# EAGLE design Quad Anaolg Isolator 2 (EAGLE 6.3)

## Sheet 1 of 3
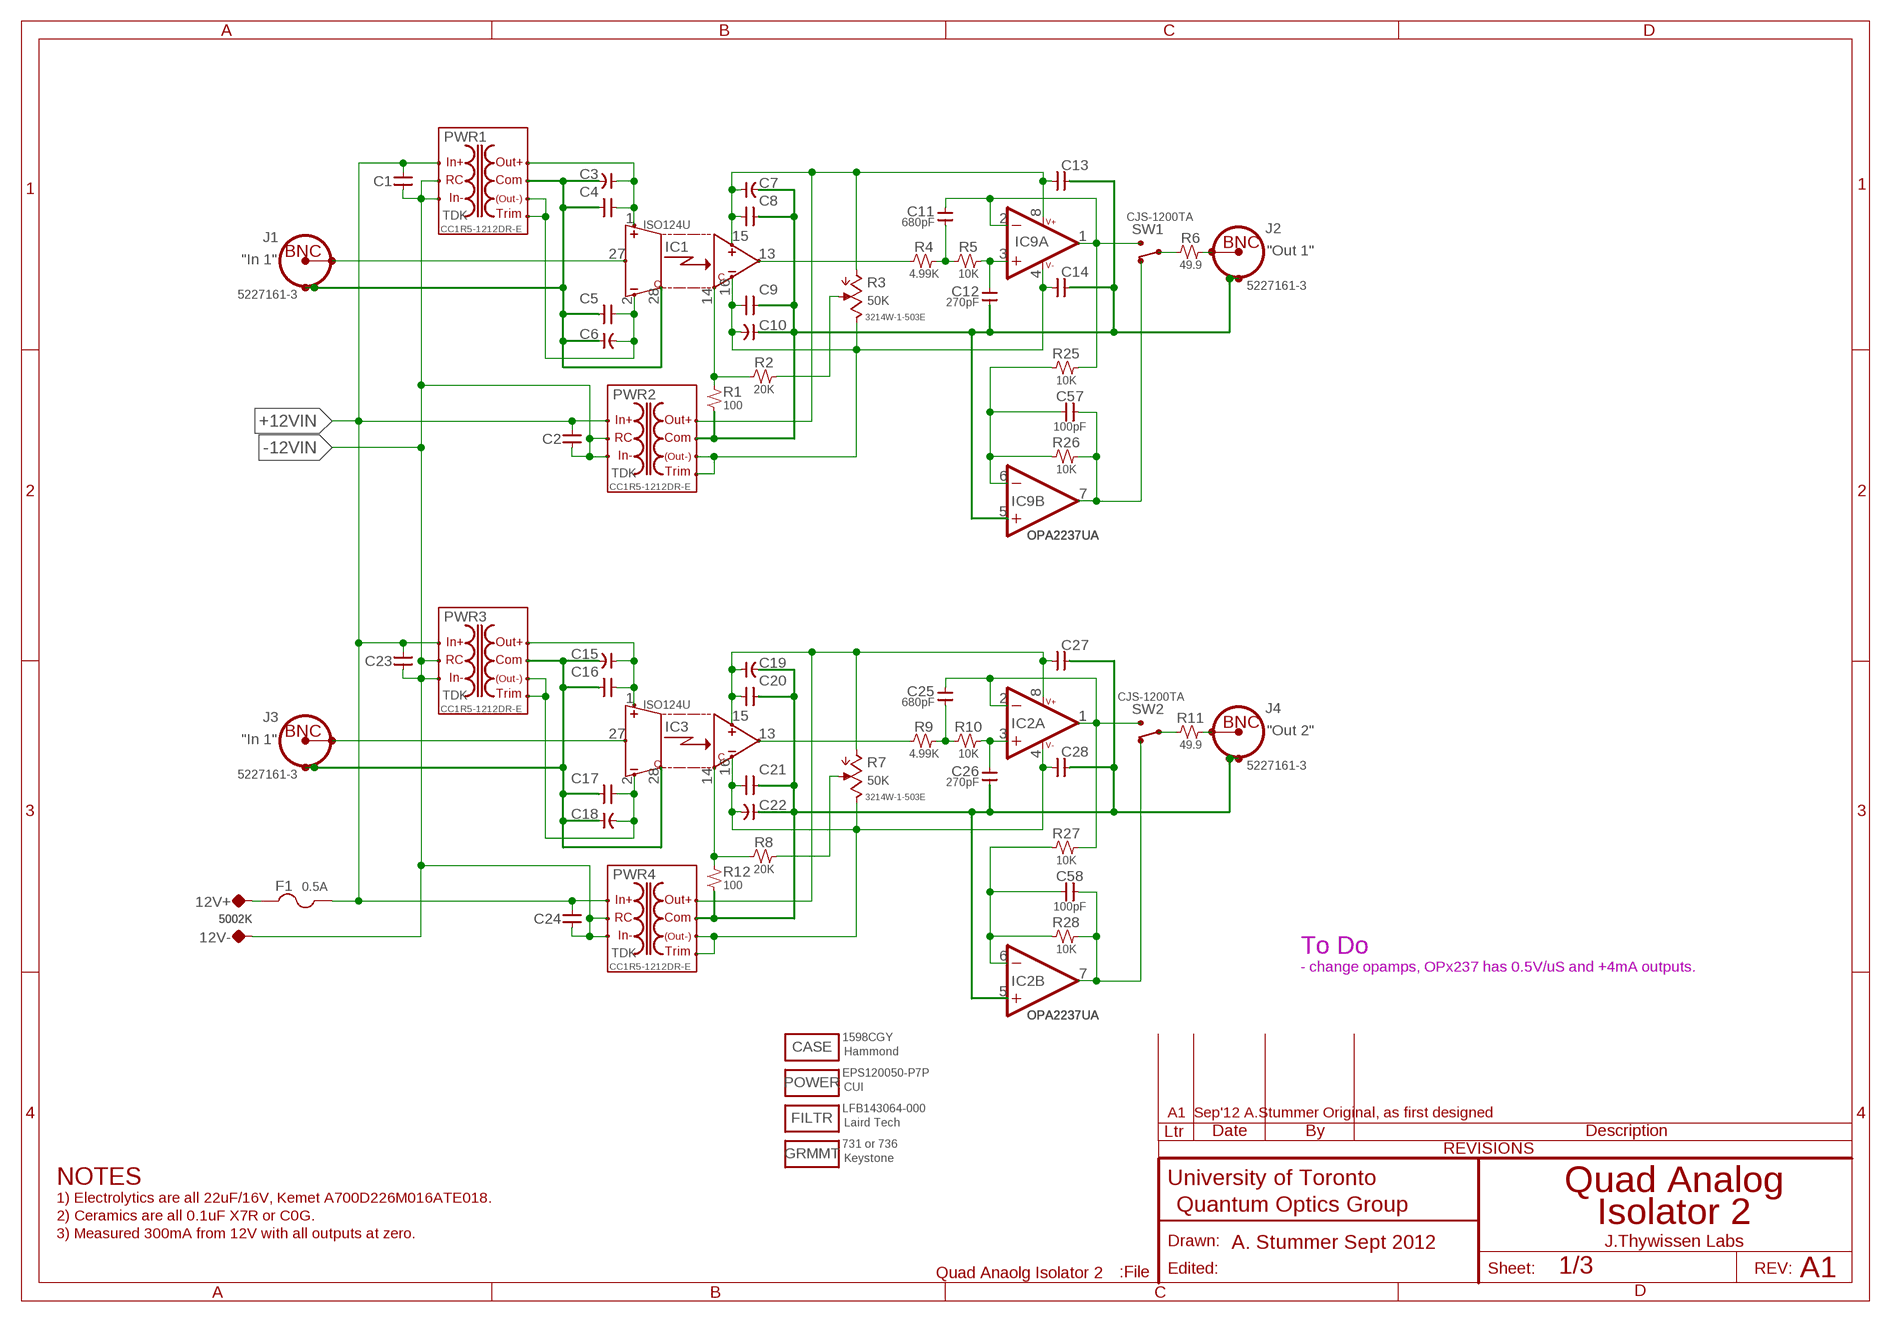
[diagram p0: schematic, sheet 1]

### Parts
12V+  5002K  TP-0.042B  [TP-0.042B]
12V-  5002K  TP-0.042B  [TP-0.042B]
C1  0.1uF  CAP-H-0805  [2012(0805)]
C2  0.1uF  CAP-H-0805  [2012(0805)]
C3  22uF  CAP-POL-2917(7343)  [2917(7343)]
C4  0.1uF  CAP-H-0805  [2012(0805)]
C5  0.1uF  CAP-H-0805  [2012(0805)]
C6  22uF  CAP-POL-2917(7343)  [2917(7343)]
C7  22uF  CAP-POL-2917(7343)  [2917(7343)]
C8  0.1uF  CAP-H-0805  [2012(0805)]
C9  0.1uF  CAP-H-0805  [2012(0805)]
C10  22uF  CAP-POL-2917(7343)  [2917(7343)]
C11  680pF  CAP-V-0805  [2012(0805)]
C12  270pF  CAP-V-0805  [2012(0805)]
C13  0.1uF  CAP-H-0805  [2012(0805)]
C14  0.1uF  CAP-H-0805  [2012(0805)]
C15  22uF  CAP-POL-SMT,8MM,PLASTIC_BASE  [CAP,POL,8MM,PLASTIC_BASE]
C16  0.1uF  CAP-H-0805  [2012(0805)]
C17  0.1uF  CAP-H-0805  [2012(0805)]
C18  22uF  CAP-POL-SMT,8MM,PLASTIC_BASE  [CAP,POL,8MM,PLASTIC_BASE]
C19  22uF  CAP-POL-SMT,8MM,PLASTIC_BASE  [CAP,POL,8MM,PLASTIC_BASE]
C20  0.1uF  CAP-H-0805  [2012(0805)]
C21  0.1uF  CAP-H-0805  [2012(0805)]
C22  22uF  CAP-POL-SMT,8MM,PLASTIC_BASE  [CAP,POL,8MM,PLASTIC_BASE]
C23  0.1uF  CAP-H-0805  [2012(0805)]
C24  0.1uF  CAP-H-0805  [2012(0805)]
C25  680pF  CAP-V-0805  [2012(0805)]
C26  270pF  CAP-V-0805  [2012(0805)]
C27  0.1uF  CAP-H-0805  [2012(0805)]
C28  0.1uF  CAP-H-0805  [2012(0805)]
C57  100pF  CAP-H-0805  [2012(0805)]
C58  100pF  CAP-H-0805  [2012(0805)]
CASE  1598CGY  MISC  [MISC]
F1  0.5A  FUSE-5X20-4  [FUSE]
FILTR  LFB143064-000  MISC  [MISC]
GRMMT  731 or 736  MISC  [MISC]
IC1  ISO124U  ANALOG:ISOLATOR_ISO12X-SOIC28B  [SOIC28B]
IC2  OPA2237UA  OPAMP:AD8___(DUAL)-SOIC-8  [SOIC-8]
IC3  ISO124U  ANALOG:ISOLATOR_ISO12X-SOIC28B  [SOIC28B]
IC9  OPA2237UA  OPAMP:AD8___(DUAL)-SOIC-8  [SOIC-8]
J1  5227161-3  CONN:BNCTYPE3HORIZ  [CONN:BNC-AMP-TYPE3HORIZ]
J2  5227161-3  CONN:BNCTYPE3HORIZ  [CONN:BNC-AMP-TYPE3HORIZ]
J3  5227161-3  CONN:BNCTYPE3HORIZ  [CONN:BNC-AMP-TYPE3HORIZ]
J4  5227161-3  CONN:BNCTYPE3HORIZ  [CONN:BNC-AMP-TYPE3HORIZ]
POWER  EPS120050-P7P  MISC  [MISC]
PWR1  CC1R5-1212DR-E  DC-DC:CCP-__-E(TDK1.5-25W)-CC1R5-R-E  [DC-DC:CC1R5-XXXXX-R-E(TDK/LAMBDA)]
PWR2  CC1R5-1212DR-E  DC-DC:CCP-__-E(TDK1.5-25W)-CC1R5-R-E  [DC-DC:CC1R5-XXXXX-R-E(TDK/LAMBDA)]
PWR3  CC1R5-1212DR-E  DC-DC:CCP-__-E(TDK1.5-25W)-CC1R5-R-E  [DC-DC:CC1R5-XXXXX-R-E(TDK/LAMBDA)]
PWR4  CC1R5-1212DR-E  DC-DC:CCP-__-E(TDK1.5-25W)-CC1R5-R-E  [DC-DC:CC1R5-XXXXX-R-E(TDK/LAMBDA)]
R1  100  R-V-0805  [2012(0805)]
R2  20K  R-H-0805  [2012(0805)]
R3  50K  POT-3214W_TRIM  [BOURNS_3214]
R4  4.99K  R-H-0805  [2012(0805)]
R5  10K  R-H-0805  [2012(0805)]
R6  49.9  R-H-0805  [2012(0805)]
R7  50K  POT-3214W_TRIM  [BOURNS_3214]
R8  20K  R-H-0805  [2012(0805)]
R9  4.99K  R-H-0805  [2012(0805)]
R10  10K  R-H-0805  [2012(0805)]
R11  49.9  R-H-0805  [2012(0805)]
R12  100  R-V-0805  [2012(0805)]
R25  10K  R-H-0805  [2012(0805)]
R26  10K  R-H-0805  [2012(0805)]
R27  10K  R-H-0805  [2012(0805)]
R28  10K  R-H-0805  [2012(0805)]
SW1  CJS-1200TA  SWITCH:SPDT_CJS-1200A1  [SWITCH:SPDT-DIP(COPAL)]
SW2  CJS-1200TA  SWITCH:SPDT_CJS-1200A1  [SWITCH:SPDT-DIP(COPAL)]

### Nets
+12VIN [isolated]: C1.2 C2.2 C23.2 C24.2 F1.2A PWR1.+VIN(+IN) PWR2.+VIN(+IN) PWR3.+VIN(+IN) PWR4.+VIN(+IN) ; also sheet 2
-12VIN [isolated]: 12V-.TP C1.1 C2.1 C23.1 C24.1 PWR1.-VIN(-IN) PWR1.RC PWR2.-VIN(-IN) PWR2.RC PWR3.-VIN(-IN) PWR3.RC PWR4.-VIN(-IN) PWR4.RC ; also sheet 2
COM-IN1 [Common]: C3.-(NEG) C4.1 C5.1 C6.+(POS) IC1.28(IN-COM) J1.SHIELD1 J1.SHIELD2 PWR1.COM
COM-IN2 [Common]: C15.NEG C16.1 C17.1 C18.POS IC3.28(IN-COM) J3.SHIELD1 J3.SHIELD2 PWR3.COM
COM-OUT1 [Common]: C7.-(NEG) C8.1 C9.1 C10.+(POS) C12.1 C13.1 C14.1 IC9.5(B:+IN) J2.SHIELD1 J2.SHIELD2 PWR2.COM R1.1
COM-OUT2 [Common]: C19.NEG C20.1 C21.1 C22.POS C26.1 C27.1 C28.1 IC2.5(B:+IN) J4.SHIELD1 J4.SHIELD2 PWR4.COM R12.1
N$1 [power]: C3.+(POS) C4.2 IC1.1(IN+V) PWR1.+VOUT(+OUT)
N$2 [power]: C5.2 C6.-(NEG) IC1.2(IN-V) PWR1.-VOUT(-OUT) PWR1.TRM(TRIM)
N$3 [power]: C15.POS C16.2 IC3.1(IN+V) PWR3.+VOUT(+OUT)
N$4 [power]: C7.+(POS) C8.2 C13.2 IC1.15(OUT+V) IC9.8(PWR:V++) PWR2.+VOUT(+OUT) R3.CCW
N$5: IC1.27(IN) J1.CONDUCTOR
N$6 [power]: C17.2 C18.NEG IC3.2(IN-V) PWR3.-VOUT(-OUT) PWR3.TRM(TRIM)
N$7: IC3.27(IN) J3.CONDUCTOR
N$8: IC1.13(OUT) R4.1
N$9: IC1.14(OUT-COM) R1.2 R2.1
N$10: R2.2 R3.W
N$11 [isolated]: 12V+.TP F1.1A
N$13 [power]: C19.POS C20.2 C27.2 IC2.8(PWR:V++) IC3.15(OUT+V) PWR4.+VOUT(+OUT) R7.CCW
N$14: J2.CONDUCTOR R6.2
N$15: IC3.13(OUT) R9.1
N$16: C11.1 R4.2 R5.1
N$17: C12.2 IC9.3(A:+IN) R5.2
N$18: C11.2 IC9.1(A:OUT) IC9.2(A:-IN) R25.2 SW1.1(NO\UP\RIGHT)
N$19 [power]: C9.2 C10.-(NEG) C14.2 IC1.16(OUT-V) IC9.4(PWR:V-) PWR2.-VOUT(-OUT) PWR2.TRM(TRIM) R3.CW
N$20: IC3.14(OUT-COM) R8.1 R12.2
N$21: R7.W R8.2
N$23: C58.1 IC2.6(B:-IN) R27.1 R28.1
N$24: C25.1 R9.2 R10.1
N$25: C26.2 IC2.3(A:+IN) R10.2
N$26: C25.2 IC2.1(A:OUT) IC2.2(A:-IN) R27.2 SW2.1(NO\UP\RIGHT)
N$27 [power]: C21.2 C22.NEG C28.2 IC2.4(PWR:V-) IC3.16(OUT-V) PWR4.-VOUT(-OUT) PWR4.TRM(TRIM) R7.CW
N$28: J4.CONDUCTOR R11.2
N$36: C58.2 IC2.7(B:OUT) R28.2 SW2.2(NC\DOWN\LEFT)
N$59: C57.1 IC9.6(B:-IN) R25.1 R26.1
N$61: C57.2 IC9.7(B:OUT) R26.2 SW1.2(NC\DOWN\LEFT)
N$62: R6.1 SW1.COM
N$63: R11.1 SW2.COM

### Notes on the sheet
- To Do
- - change opamps, OPx237 has 0.5V/uS and +4mA outputs.
- A1  Sep'12 A.Stummer Original, as first designed
- NOTES
- Quad Analog
- 1) Electrolytics are all 22uF/16V, Kemet A700D226M016ATE018.
- 2) Ceramics are all 0.1uF X7R or C0G. | Isolator 2
- 3) Measured 300mA from 12V with all outputs at zero.
- A. Stummer Sept 2012 | J.Thywissen Labs
- A1

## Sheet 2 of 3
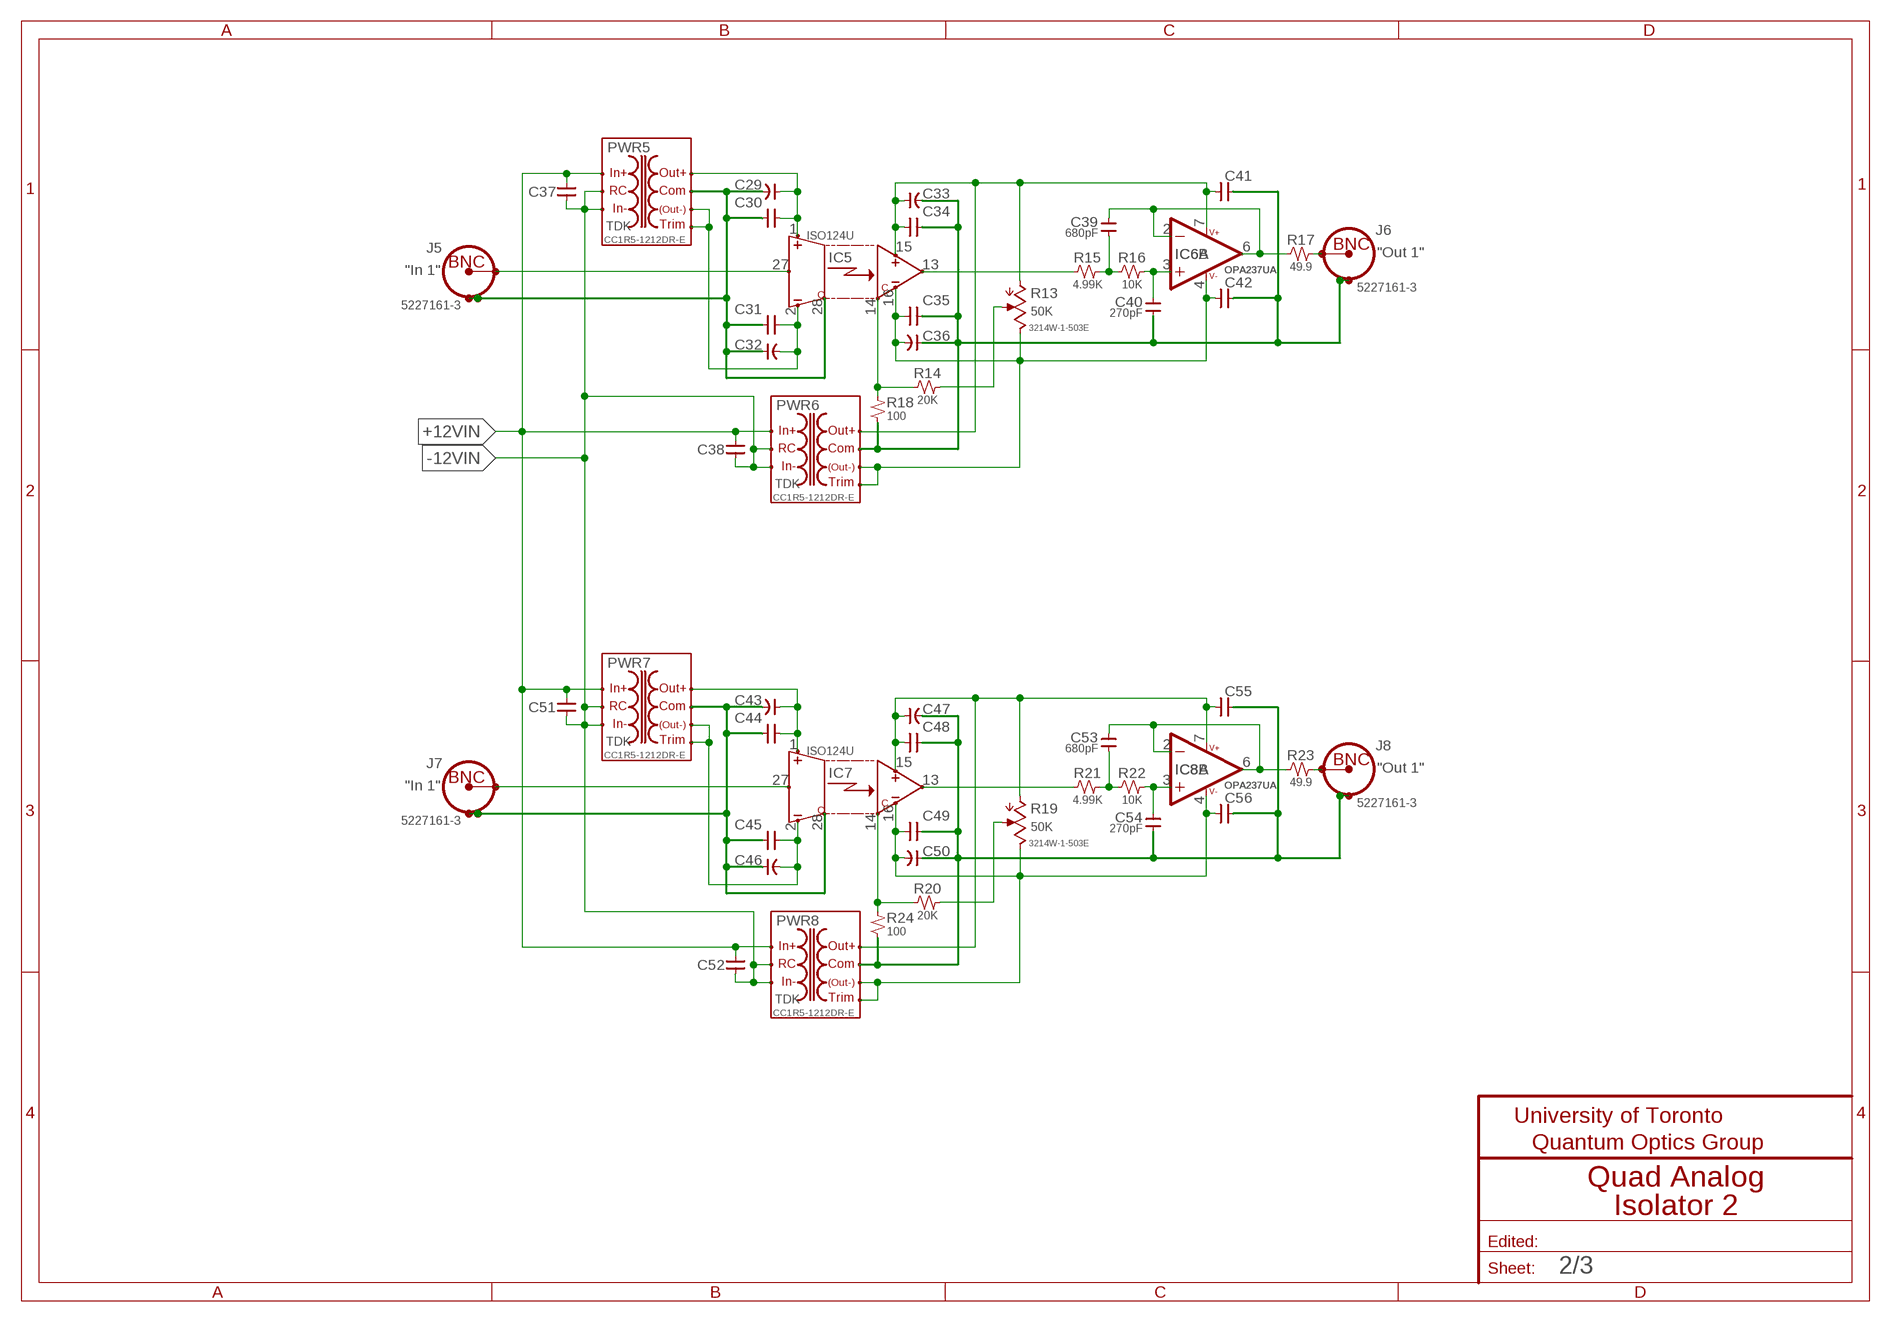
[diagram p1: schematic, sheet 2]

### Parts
C29  22uF  CAP-POL-SMT,8MM,PLASTIC_BASE  [CAP,POL,8MM,PLASTIC_BASE]
C30  0.1uF  CAP-H-0805  [2012(0805)]
C31  0.1uF  CAP-H-0805  [2012(0805)]
C32  22uF  CAP-POL-SMT,8MM,PLASTIC_BASE  [CAP,POL,8MM,PLASTIC_BASE]
C33  22uF  CAP-POL-SMT,8MM,PLASTIC_BASE  [CAP,POL,8MM,PLASTIC_BASE]
C34  0.1uF  CAP-H-0805  [2012(0805)]
C35  0.1uF  CAP-H-0805  [2012(0805)]
C36  22uF  CAP-POL-SMT,8MM,PLASTIC_BASE  [CAP,POL,8MM,PLASTIC_BASE]
C37  0.1uF  CAP-H-0805  [2012(0805)]
C38  0.1uF  CAP-H-0805  [2012(0805)]
C39  680pF  CAP-V-0805  [2012(0805)]
C40  270pF  CAP-V-0805  [2012(0805)]
C41  0.1uF  CAP-H-0805  [2012(0805)]
C42  0.1uF  CAP-H-0805  [2012(0805)]
C43  22uF  CAP-POL-SMT,8MM,PLASTIC_BASE  [CAP,POL,8MM,PLASTIC_BASE]
C44  0.1uF  CAP-H-0805  [2012(0805)]
C45  0.1uF  CAP-H-0805  [2012(0805)]
C46  22uF  CAP-POL-SMT,8MM,PLASTIC_BASE  [CAP,POL,8MM,PLASTIC_BASE]
C47  22uF  CAP-POL-SMT,8MM,PLASTIC_BASE  [CAP,POL,8MM,PLASTIC_BASE]
C48  0.1uF  CAP-H-0805  [2012(0805)]
C49  0.1uF  CAP-H-0805  [2012(0805)]
C50  22uF  CAP-POL-SMT,8MM,PLASTIC_BASE  [CAP,POL,8MM,PLASTIC_BASE]
C51  0.1uF  CAP-H-0805  [2012(0805)]
C52  0.1uF  CAP-H-0805  [2012(0805)]
C53  680pF  CAP-V-0805  [2012(0805)]
C54  270pF  CAP-V-0805  [2012(0805)]
C55  0.1uF  CAP-H-0805  [2012(0805)]
C56  0.1uF  CAP-H-0805  [2012(0805)]
IC5  ISO124U  ANALOG:ISOLATOR_ISO12X-SOIC28B  [SOIC28B]
IC6  OPA237UA  OPAMP-SO8  [SOIC-8]
IC7  ISO124U  ANALOG:ISOLATOR_ISO12X-SOIC28B  [SOIC28B]
IC8  OPA237UA  OPAMP-SO8  [SOIC-8]
J5  5227161-3  CONN:BNCTYPE3HORIZ  [CONN:BNC-AMP-TYPE3HORIZ]
J6  5227161-3  CONN:BNCTYPE3HORIZ  [CONN:BNC-AMP-TYPE3HORIZ]
J7  5227161-3  CONN:BNCTYPE3HORIZ  [CONN:BNC-AMP-TYPE3HORIZ]
J8  5227161-3  CONN:BNCTYPE3HORIZ  [CONN:BNC-AMP-TYPE3HORIZ]
PWR5  CC1R5-1212DR-E  DC-DC:CCP-__-E(TDK1.5-25W)-CC1R5-R-E  [DC-DC:CC1R5-XXXXX-R-E(TDK/LAMBDA)]
PWR6  CC1R5-1212DR-E  DC-DC:CCP-__-E(TDK1.5-25W)-CC1R5-R-E  [DC-DC:CC1R5-XXXXX-R-E(TDK/LAMBDA)]
PWR7  CC1R5-1212DR-E  DC-DC:CCP-__-E(TDK1.5-25W)-CC1R5-R-E  [DC-DC:CC1R5-XXXXX-R-E(TDK/LAMBDA)]
PWR8  CC1R5-1212DR-E  DC-DC:CCP-__-E(TDK1.5-25W)-CC1R5-R-E  [DC-DC:CC1R5-XXXXX-R-E(TDK/LAMBDA)]
R13  50K  POT-3214W_TRIM  [BOURNS_3214]
R14  20K  R-H-0805  [2012(0805)]
R15  4.99K  R-H-0805  [2012(0805)]
R16  10K  R-H-0805  [2012(0805)]
R17  49.9  R-H-0805  [2012(0805)]
R18  100  R-V-0805  [2012(0805)]
R19  50K  POT-3214W_TRIM  [BOURNS_3214]
R20  20K  R-H-0805  [2012(0805)]
R21  4.99K  R-H-0805  [2012(0805)]
R22  10K  R-H-0805  [2012(0805)]
R23  49.9  R-H-0805  [2012(0805)]
R24  100  R-V-0805  [2012(0805)]

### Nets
+12VIN [isolated]: C37.2 C38.2 C51.2 C52.2 PWR5.+VIN(+IN) PWR6.+VIN(+IN) PWR7.+VIN(+IN) PWR8.+VIN(+IN) ; also sheet 1
-12VIN [isolated]: C37.1 C38.1 C51.1 C52.1 PWR5.-VIN(-IN) PWR5.RC PWR6.-VIN(-IN) PWR6.RC PWR7.-VIN(-IN) PWR7.RC PWR8.-VIN(-IN) PWR8.RC ; also sheet 1
COM-IN3 [Common]: C29.NEG C30.1 C31.1 C32.POS IC5.28(IN-COM) J5.SHIELD1 J5.SHIELD2 PWR5.COM
COM-IN4 [Common]: C43.NEG C44.1 C45.1 C46.POS IC7.28(IN-COM) J7.SHIELD1 J7.SHIELD2 PWR7.COM
COM-OUT3 [Common]: C33.NEG C34.1 C35.1 C36.POS C40.1 C41.1 C42.1 J6.SHIELD1 J6.SHIELD2 PWR6.COM R18.1
COM-OUT4 [Common]: C47.NEG C48.1 C49.1 C50.POS C54.1 C55.1 C56.1 J8.SHIELD1 J8.SHIELD2 PWR8.COM R24.1
N$29 [power]: C29.POS C30.2 IC5.1(IN+V) PWR5.+VOUT(+OUT)
N$30 [power]: C31.2 C32.NEG IC5.2(IN-V) PWR5.-VOUT(-OUT) PWR5.TRM(TRIM)
N$31: IC5.27(IN) J5.CONDUCTOR
N$32 [power]: C33.POS C34.2 C41.2 IC5.15(OUT+V) IC6.7(B:V++) PWR6.+VOUT(+OUT) R13.CCW
N$33: IC5.13(OUT) R15.1
N$34: IC5.14(OUT-COM) R14.1 R18.2
N$35: R13.W R14.2
N$38: C39.1 R15.2 R16.1
N$39: C40.2 IC6.3(A:+IN) R16.2
N$40: C39.2 IC6.2(A:-IN) IC6.6(A:OUT) R17.1
N$41 [power]: C35.2 C36.NEG C42.2 IC5.16(OUT-V) IC6.4(B:V-) PWR6.-VOUT(-OUT) PWR6.TRM(TRIM) R13.CW
N$42: J6.CONDUCTOR R17.2
N$43 [power]: C43.POS C44.2 IC7.1(IN+V) PWR7.+VOUT(+OUT)
N$44 [power]: C45.2 C46.NEG IC7.2(IN-V) PWR7.-VOUT(-OUT) PWR7.TRM(TRIM)
N$45: IC7.27(IN) J7.CONDUCTOR
N$46 [power]: C47.POS C48.2 C55.2 IC7.15(OUT+V) IC8.7(B:V++) PWR8.+VOUT(+OUT) R19.CCW
N$47: IC7.13(OUT) R21.1
N$48: IC7.14(OUT-COM) R20.1 R24.2
N$49: R19.W R20.2
N$52: C53.1 R21.2 R22.1
N$53: C54.2 IC8.3(A:+IN) R22.2
N$54: C53.2 IC8.2(A:-IN) IC8.6(A:OUT) R23.1
N$55 [power]: C49.2 C50.NEG C56.2 IC7.16(OUT-V) IC8.4(B:V-) PWR8.-VOUT(-OUT) PWR8.TRM(TRIM) R19.CW
N$56: J8.CONDUCTOR R23.2

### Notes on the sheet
- Quad Analog
- Isolator 2

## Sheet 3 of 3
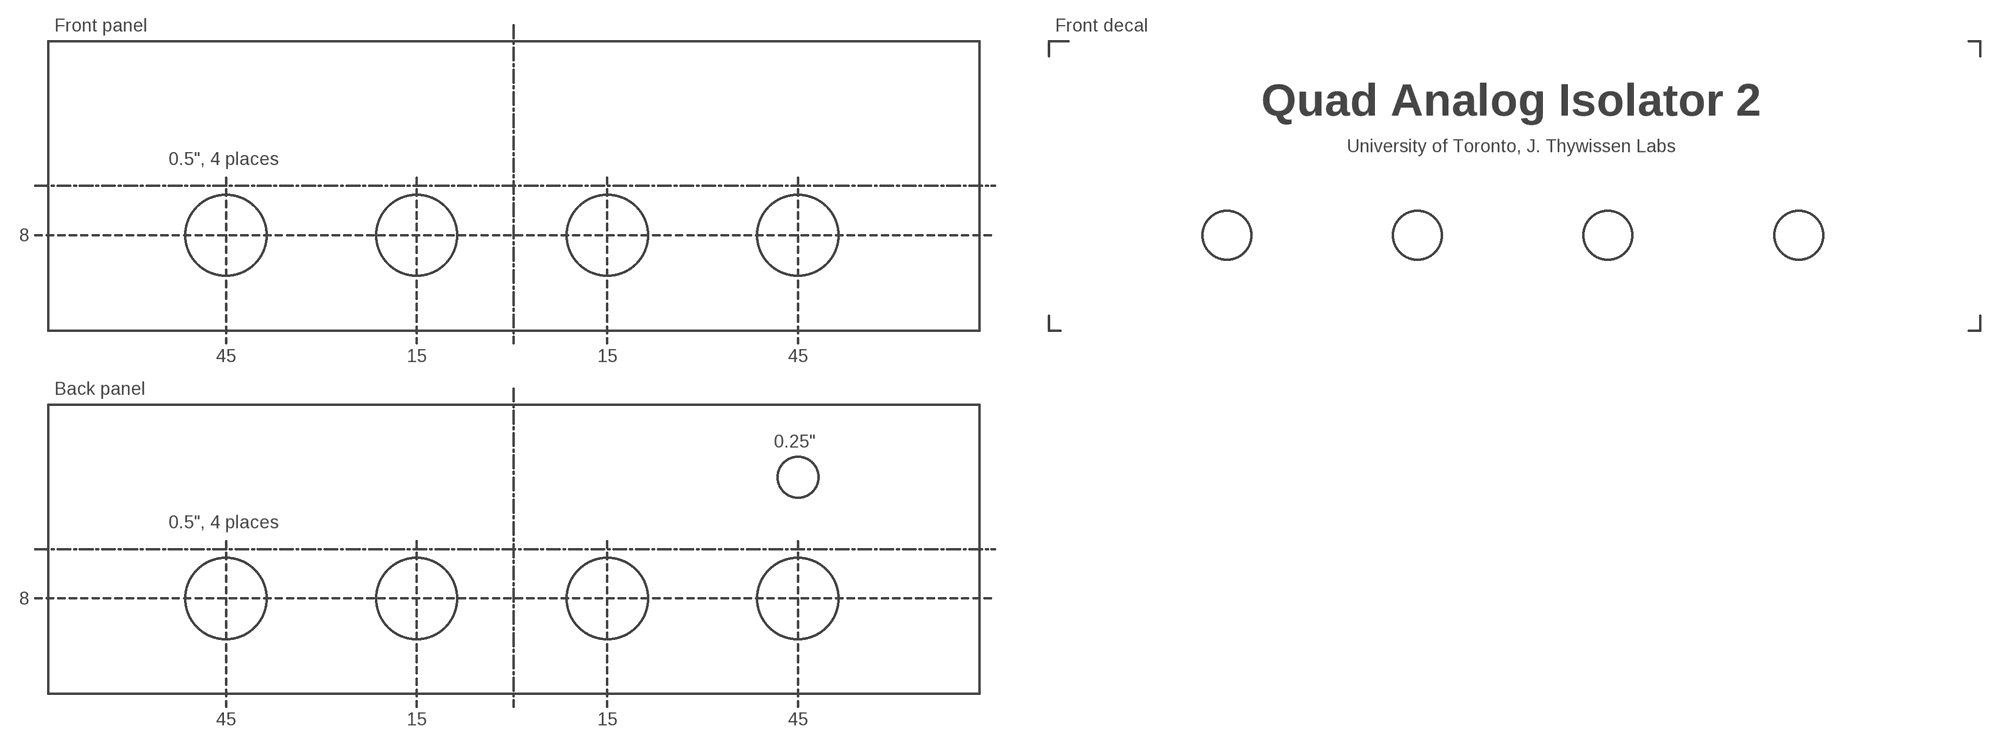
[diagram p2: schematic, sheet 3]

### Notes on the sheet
- Front panel | Front decal
- Quad Analog Isolator 2
- University of Toronto, J. Thywissen Labs
- 0.5", 4 places
- 8
- 45 | 15 | 15 | 45
- Back panel
- 0.25"
- 0.5", 4 places
- 8
- 45 | 15 | 15 | 45

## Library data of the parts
12V+ 12V- = QuantumOptics:TP: Testpoint, single pin or single socket, either SMT pad, small hole or loop style TP such as Keystone 5002K (0.042").
C1 C2 C4 C5 C8 C9 C13 C14 C16 C17 C20 C21 C23 C24 C27 C28 C30 C31 C34 C35 C37 C38 C41 C42 C44 C45 C48 C49 C51 C52 C55-C58 = QuantumOptics:CAP-H-: Cap, SMT and Through-hole, 0402 and up.
C3 C6 C7 C10 C15 C18 C19 C22 C29 C32 C33 C36 C43 C46 C47 C50 = QuantumOptics:CAP-POL-: Capacitor, Polarized, SMT 0805 and up, probably tantalum.; MFG: Kemet; PN: A700D226M016ATE018
C11 C12 C25 C26 C39 C40 C53 C54 = QuantumOptics:CAP-V-: Cap, SMT and Through-hole, 0402 and up.
CASE = QuantumOptics:MISC: Miscellaneous Part, just a placeholder for miscellaeous parts; MFG: Hammond
F1 = QuantumOptics:FUSE: Fuse; PN: 2 x 100056
FILTR = QuantumOptics:MISC: Miscellaneous Part, just a placeholder for miscellaeous parts; MFG: Laird Tech
GRMMT = QuantumOptics:MISC: Miscellaneous Part, just a placeholder for miscellaeous parts; MFG: Keystone
IC1 IC3 IC5 IC7 = QuantumOptics:ANALOG:ISOLATOR_ISO12X: Analog Isolator, ISO12x T.I., ±10V gain=1. http://focus.ti.com/lit/ds/symlink/iso124.pdf
IC2 IC9 = QuantumOptics:OPAMP:AD8___(DUAL): AD8xxx, Analog Devices, dual opamp in SOIC-8 and MSOP-8, various versions available. AD8066, AD8656, etc. e.g. http://www.analog.com/UploadedFiles/Data_Sheets/476080131AD8655_6_a.pdf
IC6 IC8 = QuantumOptics:OPAMP: Op Amp, generic, pick the right package. e.g. AD8605: SOT-23-5, RRIO, 10MHz, Ib = 1pA, Vio < 65uV, 2.7-5.5V.
J1 J3 J5 J7 = QuantumOptics:CONN:BNC: BNC PCB, horizontal or vertical, e.g. Horiz: Amp (5)227677-1, nut 1-329631-2, shoulder washer 330620, vert isolated 5227222-6, http://catalog.tycoelectronics.com/TE/bin/TE.Connect?C=1&M=BYPN&TCPN=5227222-6&RQPN=5227222-6 ...; DESC: "In 1"
J2 J6 J8 = QuantumOptics:CONN:BNC: BNC PCB, horizontal or vertical, e.g. Horiz: Amp (5)227677-1, nut 1-329631-2, shoulder washer 330620, vert isolated 5227222-6, http://catalog.tycoelectronics.com/TE/bin/TE.Connect?C=1&M=BYPN&TCPN=5227222-6&RQPN=5227222-6 ...; DESC: "Out 1"
J4 = QuantumOptics:CONN:BNC: BNC PCB, horizontal or vertical, e.g. Horiz: Amp (5)227677-1, nut 1-329631-2, shoulder washer 330620, vert isolated 5227222-6, http://catalog.tycoelectronics.com/TE/bin/TE.Connect?C=1&M=BYPN&TCPN=5227222-6&RQPN=5227222-6 ...; DESC: "Out 2"
POWER = QuantumOptics:MISC: Miscellaneous Part, just a placeholder for miscellaeous parts; MFG: CUI
PWR1-PWR8 = QuantumOptics:DC-DC:CCP-__-E(TDK1.5-25W): CCp-inoutsc-E, TDK DC-DC isolated, 1.5-25W, uni- or bipolar "p": 1.5, 3, 6, 10, 15, or 25W. "in": Input 05, 12, 24 or 48V. "out": Output 3.3, 5, 12, ±12 (or 24), ±15 (or30V). "s": Polarity single or dual. "c": Case horiz DIP, horiz SMD or vertical SIP. http://www.tdk.co.jp/tefe02/ea335_cc_e.pdf
R1 R12 R18 R24 = QuantumOptics:R-V-*: Resistor, SMT & Through-Hole, vertical symbol
R2 R4-R6 R8-R11 R14-R17 R20-R23 R25-R28 = QuantumOptics:R-H-*: Resistor, SMT & Through-Hole, horizontal symbol
R3 R7 R13 R19 = QuantumOptics:POT: Pot, regular or trimpot; PN: 3214W-1-503E
SW1 SW2 = QuantumOptics:SWITCH:SPDT: Switch, SPDT

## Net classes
1 Common: width 0.5 mm, drill 0.711 mm
2 power: width 0.4 mm, drill 0.711 mm
3 isolated: width 0.5 mm, drill 0.711 mm, clearance 0.4 mm

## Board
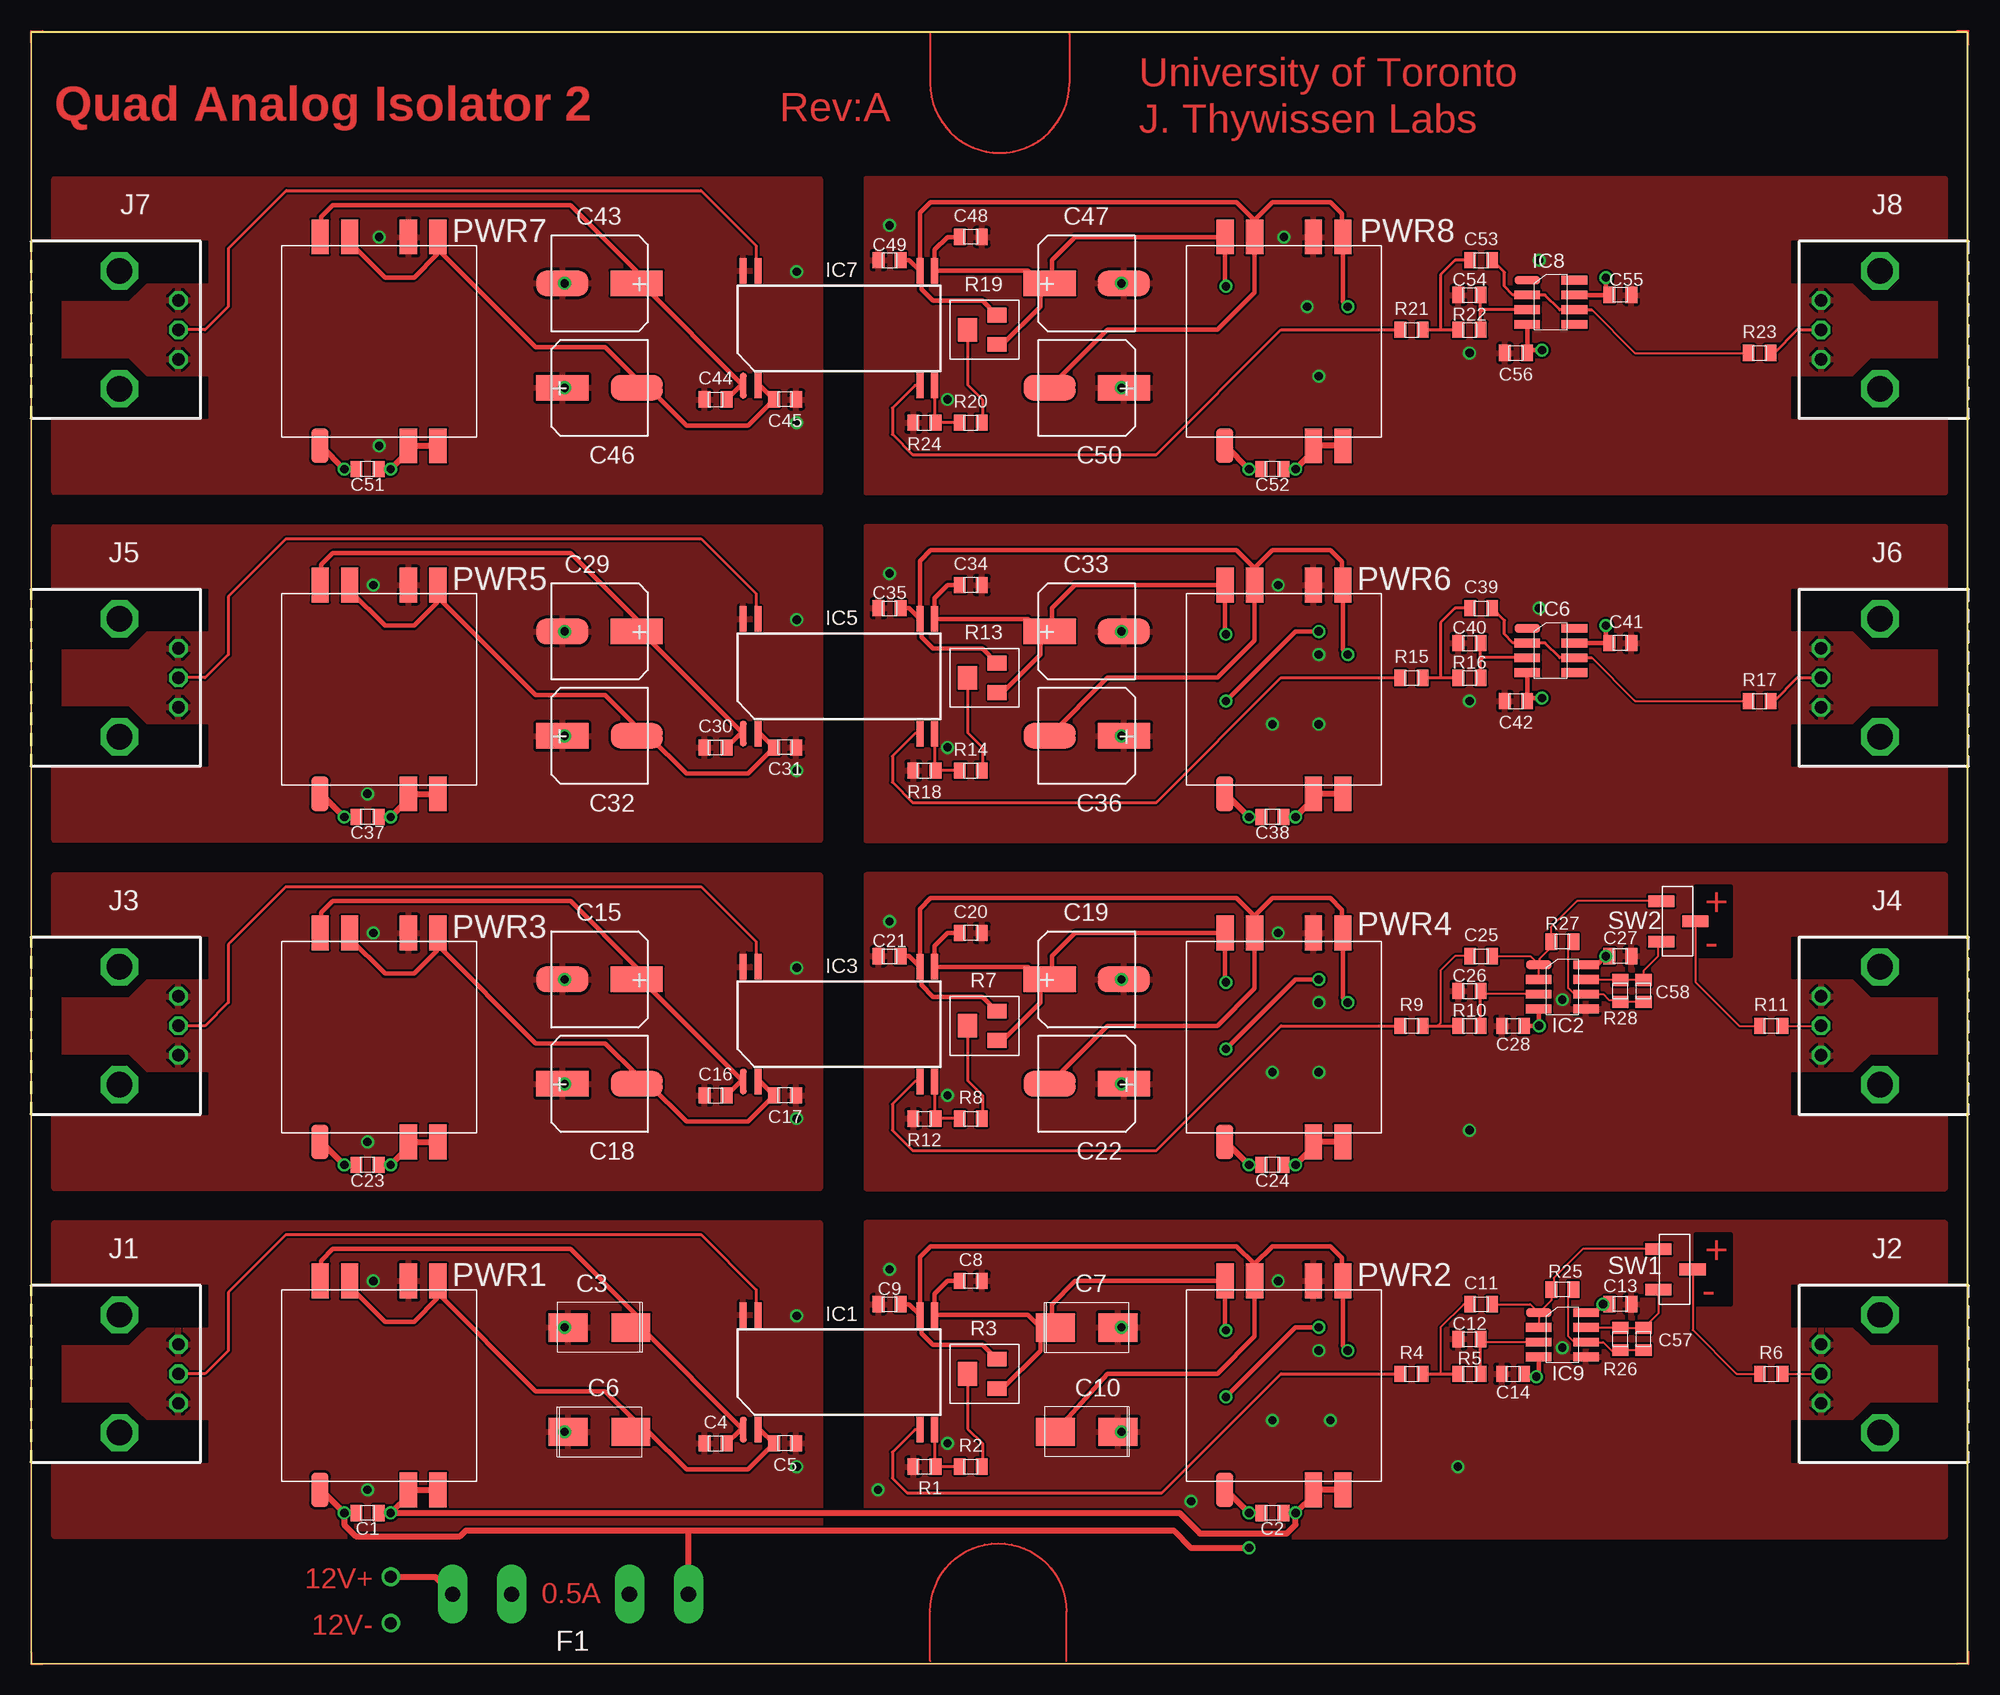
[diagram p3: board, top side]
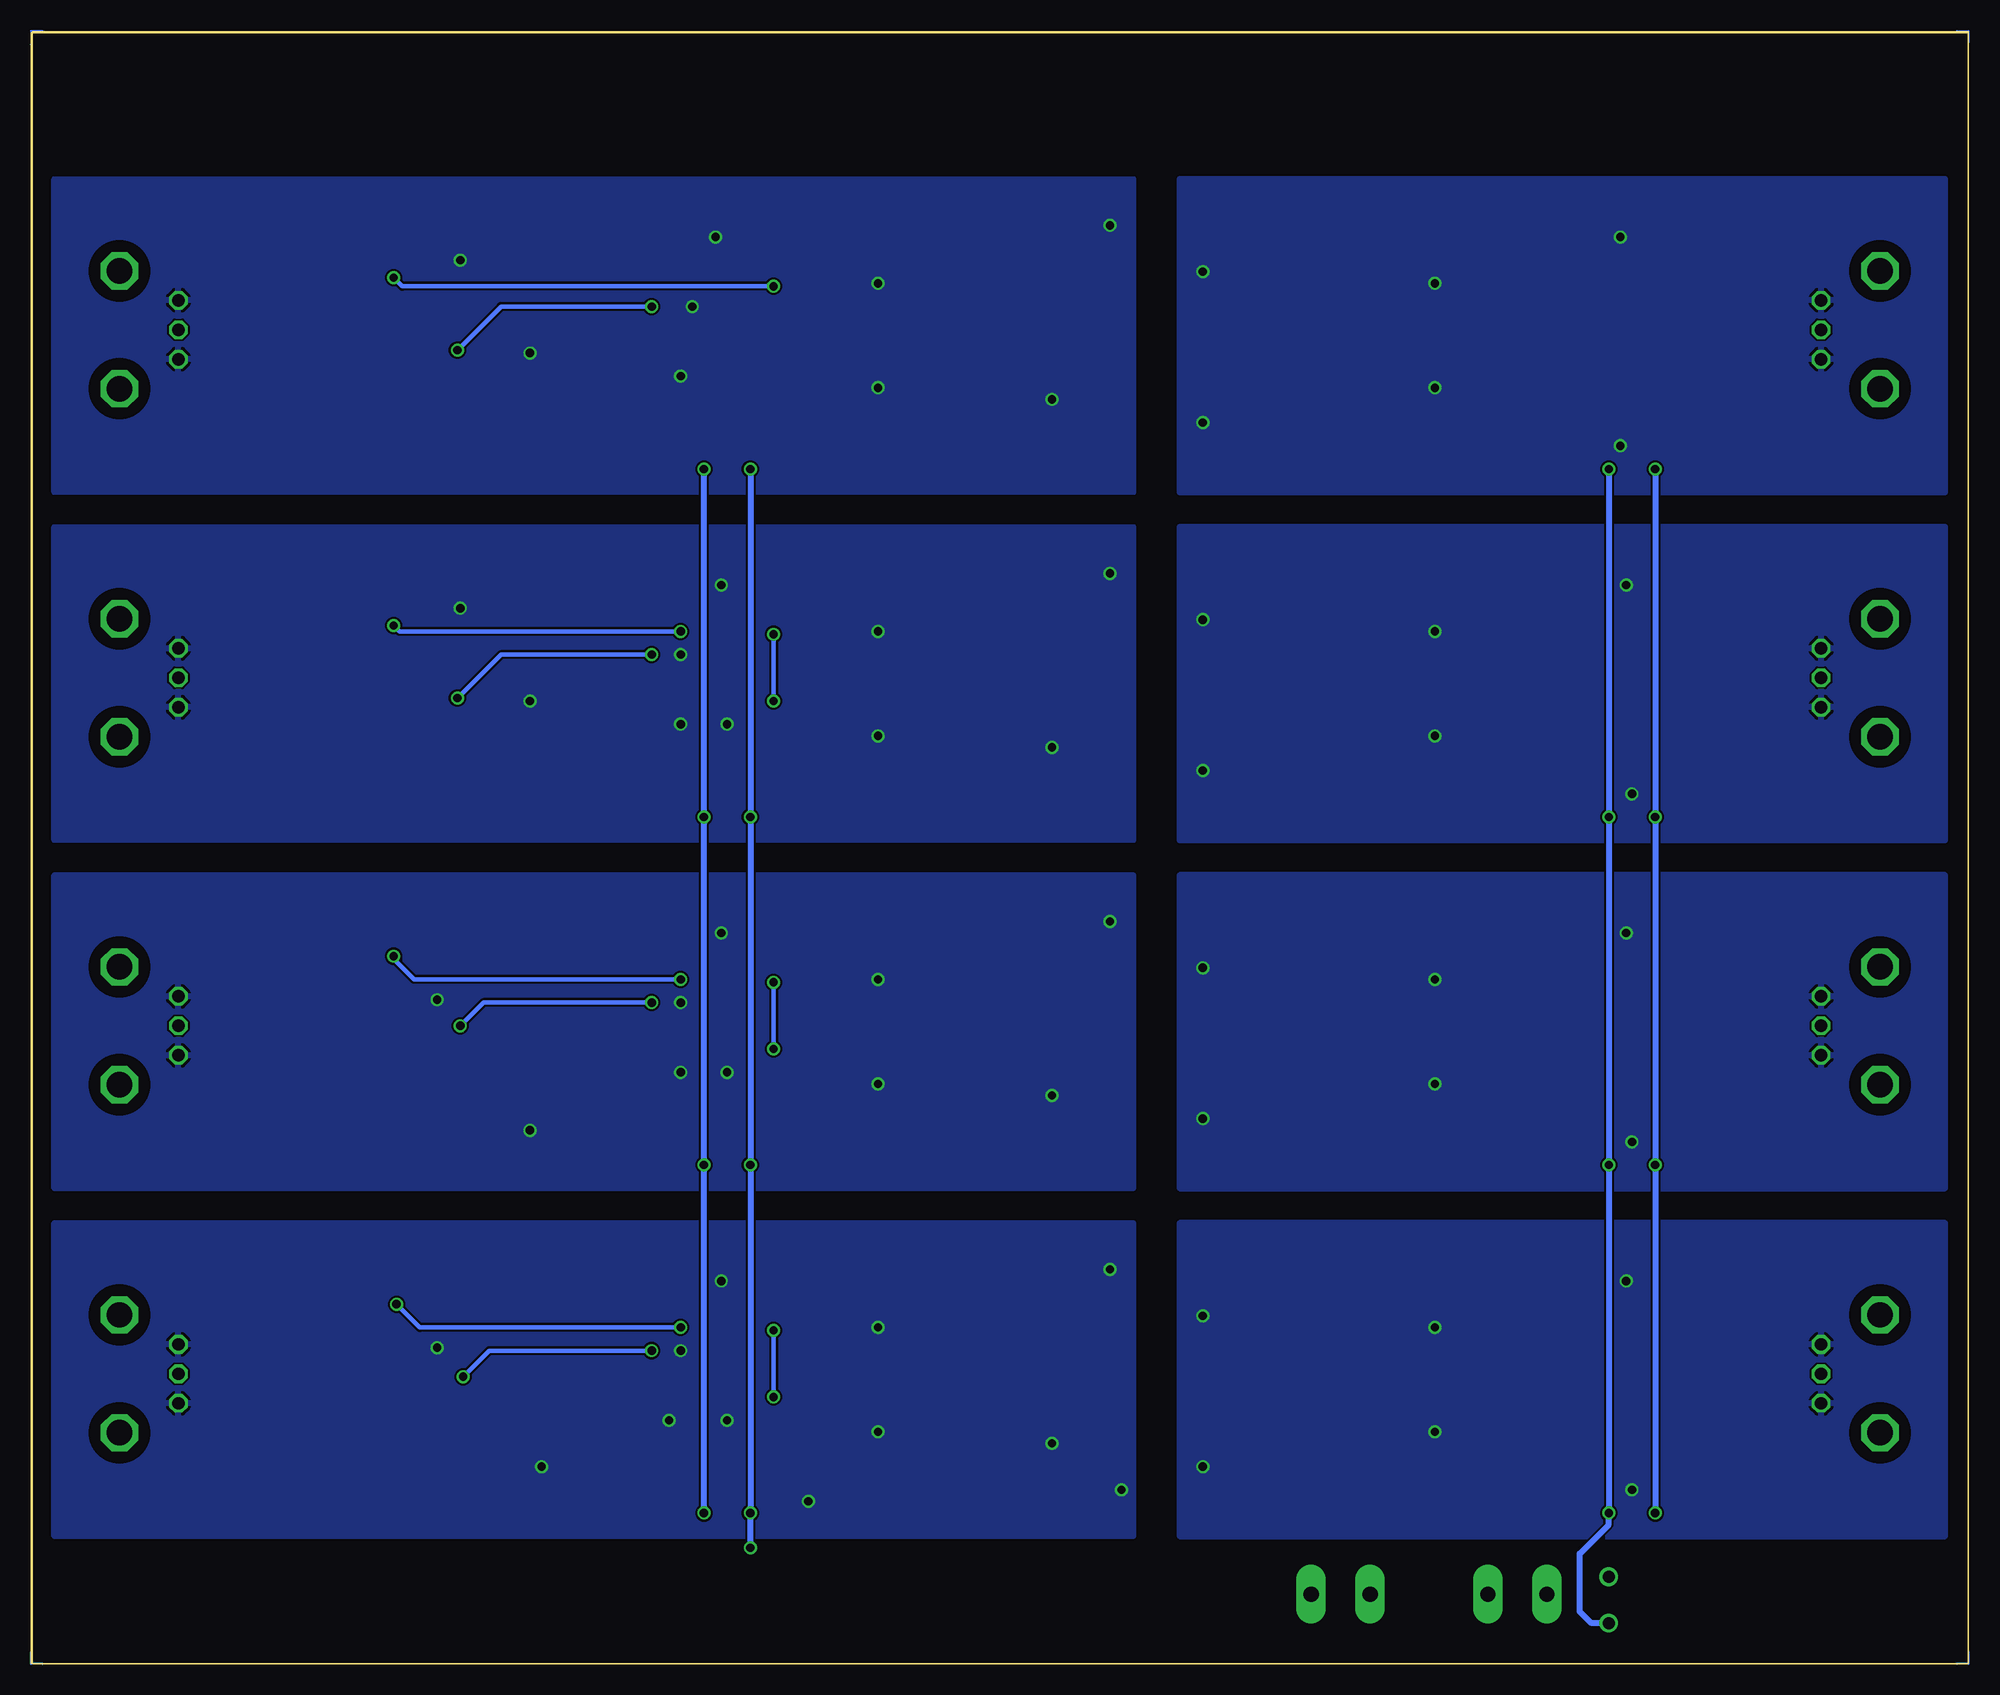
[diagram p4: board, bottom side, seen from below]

Size 167 x 140.7 mm. Coordinates in mm from the lower left corner, seen from the top.
Outline: 0,0 167,0 167,140.6 0,140.6 0,0
Copper layers (1+16): Top 0.035mm / dielectric 1.5mm / Bottom 0.035mm
Design rules "default": minimum track width 7mil, minimum drill 20mil, track to track 7mil, track to pad 7mil, pad to pad 7mil, via to via 7mil, smd to smd 0mil, copper to edge 25mil, drill to drill 8mil, minimum pad ring 10mil, minimum via ring 8mil, stop-mask expansion 4mil, vias tented up to drill 0mil, thermal gap 10mil
tRestrict: 8 lines

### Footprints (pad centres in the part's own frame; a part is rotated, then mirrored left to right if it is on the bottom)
TP-0.042B = drill 1.067: TP 0,0
2012(0805) = smd 1.016 x 1.397: 1 -0.953,0; 2 0.953,0
2917(7343) = smd 3.35 x 2.45: + -2.7,0; - 2.7,0
CAP,POL,8MM,PLASTIC_BASE = smd 4.5 x 2.2: NEG -3.2,0; POS 3.2,0
FUSE = drill 1.321 pad 2.54 long: 1A -10.16,0; 1B -5.08,0; 2A 10.16,0; 2B 5.08,0
SOIC28B = smd 0.6 x 2.2: 1 -7.62,-4.81; 2 -6.35,-4.81; 13 7.62,-4.81; 14 8.89,-4.81; 15 8.89,5.08; 16 7.62,5.08; 27 -6.35,5.08; 28 -7.62,5.08
SOIC-8 = smd 0.75 x 2.2: 1 -1.27,-2.032; 2 0,-2.032; 3 1.27,-2.032; 4 2.54,-2.032; 5 2.54,2.032; 6 1.27,2.032; 7 0,2.032; 8 -1.27,2.032
CONN:BNC-AMP-TYPE3HORIZ = drill 1.067 octagon: CONDUCTOR 0,-12.7; SHIELD1 -2.54,-12.7; SHIELD2 2.54,-12.7 | drill 2.184 octagon: P$1 -5.08,-7.62; P$2 5.08,-7.62
DC-DC:CC1R5-XXXXX-R-E(TDK/LAMBDA) = smd 3 x 1.5: +VIN -9,5.1; +VOUT 9,5.08; -VIN -9,-5.08; -VOUT 9,-5.08; COM 9,-2.54; RC -9,-2.54; TRM 9,2.54
BOURNS_3214 = smd 1.651 x 1.27: CCW 1.27,-1.27; CW 1.27,1.27 | smd 1.651 x 2.032: W -1.27,0
SWITCH:SPDT-DIP(COPAL) = smd 1 x 2.25: 1 -1.75,-1.475; 2 1.75,-1.475; COM 0,1.475

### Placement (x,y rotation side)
12V+  31,7.5 180 top
12V-  31,3.5 180 top
C1  29,13 180 top
C2  107,13 180 top
C3  49,29 180 top
C4  59,19 0 top
C5  65,19 180 top
C6  49,20 0 top
C7  91,29 0 top
C8  81,33 180 top
C9  74,31 0 top
C10  91,20 180 top
C11  125,31 0 top
C12  124,28 0 top
C13  137,31 180 top
C14  127.75,25 0 top
C15  49,59 0 top
C16  59,49 0 top
C17  65,49 180 top
C18  49,50 180 top
C19  91,59 180 top
C20  81,63 180 top
C21  74,61 0 top
C22  91,50 0 top
C23  29,43 180 top
C24  107,43 180 top
C25  125,61 0 top
C26  124,58 0 top
C27  137,61 180 top
C28  127.75,55 0 top
C29  49,89 0 top
C30  59,79 0 top
C31  65,79 180 top
C32  49,80 180 top
C33  91,89 180 top
C34  81,93 180 top
C35  74,91 0 top
C36  91,80 0 top
C37  29,73 180 top
C38  107,73 180 top
C39  125,91 0 top
C40  124,88 0 top
C41  137,88 180 top
C42  128,83 0 top
C43  49,119 0 top
C44  59,109 0 top
C45  65,109 180 top
C46  49,110 180 top
C47  91,119 180 top
C48  81,123 180 top
C49  74,121 0 top
C50  91,110 0 top
C51  29,103 180 top
C52  107,103 180 top
C53  125,121 0 top
C54  124,118 0 top
C55  137,118 180 top
C56  128,113 0 top
C57  139,28 90 top
C58  139,58 90 top
CASE  102,-3 0 top
F1  46.5,6 0 top
FILTR  not placed on the board
GRMMT  not placed on the board
IC1  69,25 0 top
IC2  132,59 270 top
IC3  69,55 0 top
IC5  69,85 0 top
IC6  131,88 270 top
IC7  69,115 0 top
IC8  131,118 270 top
IC9  132,29 270 top
J1  0,25 90 top
J2  167,25 270 top
J3  0,55 90 top
J4  167,55 270 top
J5  0,85 90 top
J6  167,85 270 top
J7  0,115 90 top
J8  167,115 270 top
POWER  not placed on the board
PWR1  30,24 90 top
PWR2  108,24 90 top
PWR3  30,54 90 top
PWR4  108,54 90 top
PWR5  30,84 90 top
PWR6  108,84 90 top
PWR7  30,114 90 top
PWR8  108,114 90 top
R1  77,17 0 top
R2  81,17 0 top
R3  82,25 0 top
R4  119,25 0 top
R5  124,25 0 top
R6  150,25 0 top
R7  82,55 0 top
R8  81,47 0 top
R9  119,55 0 top
R10  124,55 0 top
R11  150,55 0 top
R12  77,47 0 top
R13  82,85 0 top
R14  81,77 0 top
R15  119,85 0 top
R16  124,85 0 top
R17  149,83 0 top
R18  77,77 0 top
R19  82,115 0 top
R20  81,107 0 top
R21  119,115 0 top
R22  124,115 0 top
R23  149,113 0 top
R24  77,107 0 top
R25  132,32.25 180 top
R26  137,28 90 top
R27  132,62.25 180 top
R28  137,58 90 top
SW1  141.75,34 270 top
SW2  142,64 270 top
U$1  [CASE:HAMMOND_1598C]  0,0 0 top
U$3  [TITLEBLOCK_PCB]  0,-2 0 top

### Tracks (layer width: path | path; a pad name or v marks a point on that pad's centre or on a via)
+12VIN  (via drill 0.71)
  Top 0.5: C51.2 v27,103 25,105 PWR7.+VIN | C37.2 v27,73 25,75 PWR5.+VIN | C23.2 v27,43 25,45 PWR3.+VIN | v27,13 C1.2 | PWR1.+VIN 25,15 v27,13 | C52.2 v105,103 103,105 PWR8.+VIN | C38.2 v105,73 103,75 PWR6.+VIN | C24.2 v105,43 103,45 PWR4.+VIN | C2.2 v105,13 103,15 PWR2.+VIN | v27,13 27,12 28,11 37,11 37.5,11.5 56.5,11.5 | 56.5,11.5 98.5,11.5 100,10 v105,10 | F1.2A 56.66,11.34 56.5,11.5
  Bottom 0.5: v27,103 v27,73 v27,43 v27,13 | v105,103 v105,73 v105,43 v105,13 v105,10
-12VIN  (via drill 0.71)
  Top 0.5: PWR2.-VIN PWR2.RC 110.54,14.54 v109,13 | PWR1.-VIN PWR1.RC 32.54,14.54 v31,13 | PWR4.-VIN PWR4.RC 110.54,44.54 v109,43 C24.1 | PWR3.-VIN PWR3.RC 32.54,44.54 v31,43 C23.1 | PWR6.-VIN PWR6.RC 110.54,74.54 v109,73 C38.1 | PWR5.-VIN PWR5.RC 32.54,74.54 v31,73 C37.1 | PWR8.-VIN PWR8.RC 110.54,104.54 v109,103 C52.1 | PWR7.-VIN PWR7.RC 32.54,104.54 v31,103 C51.1 | v31,13 C1.1 | v109,13 C2.1 108,12.95 | v31,13 99,13 100.75,11.25 108.25,11.25 109,12 v109,13
  Bottom 0.5: v31,103 v31,73 v31,43 v31,13 31,12 33.5,9.5 33.5,4.5 32.5,3.5 12V-.TP | v109,13 v109,43 v109,73 v109,103
COM-IN1  (via drill 0.71)
  other vias: 29.5,33 29,15 46,20 46,29 66,30 66,17
  pour Top: 2,38 68,38 68,11 2,11
  pour Bottom: 2,38 68,38 68,11 2,11
COM-IN2  (via drill 0.71)
  other vias: 29.5,63 29,45 46,50 46,59 66,60 66,47
  pour Top: 2,68 68,68 68,41 2,41
  pour Bottom: 2,68 68,68 68,41 2,41
COM-IN3  (via drill 0.71)
  other vias: 29.5,93 29,75 46,80 46,89 66,90 66,77
  pour Top: 2,98 68,98 68,71 2,71
  pour Bottom: 2,98 68,98 68,71 2,71
COM-IN4  (via drill 0.71)
  other vias: 30,123 30,105 46,110 46,119 66,120 66,107
  pour Top: 2,128 68,128 68,101 2,101
  pour Bottom: 2,128 68,128 68,101 2,101
COM-OUT1  (via drill 0.71)
  other vias: 74,34 79,19 94,20 94,29 123,17 132,27.25 111,27 112,21 107.5,33 73,15 100,14 107,21
  pour Top: 165,38 72,38 72,11 165,11
  pour Bottom: 165,38 72,38 72,11 165,11
COM-OUT2  (via drill 0.71)
  other vias: 74,64 79,49 94,50 94,59 124,46 132,57.25 111,57 111,51 107.5,63 107,51
  pour Top: 165,68 72,68 72,41 165,41
  pour Bottom: 165,68 72,68 72,41 165,41
COM-OUT3  (via drill 0.71)
  other vias: 74,94 79,79 94,80 94,89 124,83 130,91 111,87 111,81 107.5,93 107,81
  pour Top: 165,98 72,98 72,71 165,71
  pour Bottom: 165,98 72,98 72,71 165,71
COM-OUT4  (via drill 0.71)
  other vias: 74,124 79,109 94,110 94,119 124,113 130,121 110,117 111,111 108,123
  pour Top: 165,128 72,128 72,101 165,101
  pour Bottom: 165,128 72,128 72,101 165,101
N$1
  Top 0.4: C4.2 61.14,20.19 IC1.1 52.57,29 C3.+ 52.2,30.05 46.5,35.75 26,35.75 25,34.75 25,33.08 PWR1.+VOUT
N$2
  Top 0.4: IC1.2 62.86,20.19 C5.2 61.8,16.75 56.5,16.75 53.25,20 C6.- 52.2,20.8 49.5,23.5 43.5,23.5 35,32 | 27.46,33.46 PWR1.TRM 27.46,32.54 30.5,29.5 33,29.5 35,31.5 35,32 | 35,32 35,32.92 PWR1.-VOUT
N$3
  Top 0.4: C16.2 61.14,50.19 IC3.1 52.57,59 C15.POS 52.2,60.05 46.5,65.75 26,65.75 25,64.75 25,63.08 PWR3.+VOUT
N$4  (via drill 0.71)
  Top 0.4: R3.CCW 83.29,23.75 83.75,23.75 87,27 87,28.2 87.4,28.6 | 87.4,28.6 C7.+ 88,29.2 88,31 90,33 PWR2.+VOUT 102.92,28.83 v103,28.75 | 87.4,28.6 85.92,30.08 IC1.15 77.89,31.89 79,33 C8.2 | v103,23 109,29 v111,29 | IC9.8 134.77,30.27 v135.5,31 C13.2
  Bottom 0.4: v103,28.75 v103,23 | v111,29 133.5,29 v135.5,31
N$5
  Top 0.254: IC1.27 62.5,30.23 62.5,32.25 57.75,37 22,37 17,32 17,27 15,25 J1.CONDUCTOR
N$6
  Top 0.4: IC3.2 62.86,50.19 C17.2 61.8,46.75 56.5,46.75 53.25,50 C18.NEG 52.2,50.8 49.5,53.5 43.5,53.5 35,62 | 27.46,63.46 PWR3.TRM 27.46,62.54 30.5,59.5 33,59.5 35,61.5 35,62 | 35,62 35,62.92 PWR3.-VOUT
N$7
  Top 0.254: IC3.27 62.5,60.23 62.5,62.25 57.75,67 22,67 17,62 17,57 15,55 J3.CONDUCTOR
N$8
  Top 0.254: IC1.13 76.19,20.19 74.25,18.25 74.25,16 75.5,14.75 97.5,14.75 107.75,25 R4.1
N$9
  Top 0.254: R2.1 R1.2 77.89,17.06 IC1.14
N$10
  Top 0.254: R3.W 80.73,20.27 82,19 82,17.05 R2.2
N$11
  Top 0.5: 12V+.TP 34.84,7.5 F1.1A
N$12
  Top 0.178: 167,1 167,0 166,0
N$13  (via drill 0.71)
  Top 0.4: R7.CCW 83.29,53.75 83.75,53.75 87,57 87,58.2 87.4,58.6 | 87.4,58.6 C19.POS 88,59.2 88,61 90,63 PWR4.+VOUT 102.92,58.83 v103,58.75 | 87.4,58.6 85.92,60.08 IC3.15 77.89,61.89 79,63 C20.2 | v103,53 109,59 v111,59 | IC2.8 135.02,60.27 v135.75,61 C27.2
  Bottom 0.4: v103,58.75 v103,53 | v111,59 134,59 135.75,60.75 v135.75,61
N$14
  Top 0.178: R6.2 J2.CONDUCTOR
N$15
  Top 0.254: IC3.13 76.19,50.19 74.25,48.25 74.25,46 76,44.25 97,44.25 107.75,55 R9.1
N$16
  Top 0.178: C11.1 123.5,31 121.5,29 121.5,25
  Top 0.254: R4.2 121.5,25 R5.1
N$17
  Top 0.178: IC9.3 125.22,27.73 C12.2
  Top 0.254: R5.2 C12.2
N$18
  Top 0.178: IC9.1 IC9.2 | C11.2 129.24,31 IC9.1 | IC9.1 131.05,31.35 R25.2 131.25,32.45 131.25,33.25 133.75,35.75 SW1.1
N$19  (via drill 0.71)
  Top 0.4: C9.2 75.7,31 IC1.16 | 105.46,34.46 PWR2.TRM 105.46,28.21 102.25,25 92.8,25 C10.- | 105.46,34.46 107,36 112,36 113,35 113,33.08 PWR2.-VOUT 113.08,27.42 v113.5,27 | R3.CW 83.23,26.27 82,27.5 77.75,27.5 76.75,28.5 76.75,29.95 IC1.16 | 105.46,34.46 103.92,36 77.54,36 76.62,35.08 IC1.16 | C14.2 128.95,24.75 v129.75,24.75 129.97,24.97 IC9.4
  Bottom 0.4: v113.5,27 127.5,27 v129.75,24.75
N$20
  Top 0.254: R8.1 R12.2 77.89,47.06 IC3.14
N$21
  Top 0.254: R7.W 80.73,50.27 82,49 82,47.05 R8.2
N$22
  Top 0.178: 167,139.6 167,140.75 166,140.75
N$23
  Top 0.178: C58.1 R28.1 136.8,57.25 136,57.25 135.52,57.73 IC2.6 133.02,57.73 132.5,58.25 132.5,61.8 R27.1
N$24
  Top 0.178: C25.1 122.75,61 121.5,59.75 121.5,55.25 121.25,55
  Top 0.254: R9.2 121.25,55 R10.1
N$25
  Top 0.178: IC2.3 125.22,57.73 C26.2
  Top 0.254: R10.2 C26.2
N$26
  Top 0.178: IC2.2 IC2.1 | IC2.1 130,60.3 130,60.75 131.05,61.8 R27.2 131,62.3 131,63.5 133.25,65.75 SW2.1 | C25.2 129.24,61 IC2.1
N$27  (via drill 0.71)
  Top 0.4: C21.2 75.7,61 IC3.16 | 105.46,64.46 PWR4.TRM 105.46,58.21 102.25,55 92.8,55 C22.NEG | 105.46,64.46 107,66 112,66 113,65 113,63.08 PWR4.-VOUT 113.08,57.42 v113.5,57 | R7.CW 83.23,56.27 82,57.5 77.75,57.5 76.75,58.5 76.75,59.95 IC3.16 | 105.46,64.46 103.92,66 77.54,66 76.62,65.08 IC3.16 | C28.2 v130,55 129.97,55.03 IC2.4
  Bottom 0.4: v113.5,57 128,57 v130,55
N$28
  Top 0.178: R11.2 J4.CONDUCTOR
N$29
  Top 0.4: C30.2 61.14,80.19 IC5.1 52.57,89 C29.POS 52.2,90.05 46.5,95.75 26,95.75 25,94.75 25,93.08 PWR5.+VOUT
N$30
  Top 0.4: IC5.2 62.86,80.19 C31.2 61.8,76.75 56.5,76.75 53.25,80 C32.NEG 52.2,80.8 49.5,83.5 43.5,83.5 35,92 | 27.46,93.46 PWR5.TRM 27.46,92.54 30.5,89.5 33,89.5 35,91.5 35,92 | 35,92 35,92.92 PWR5.-VOUT
N$31
  Top 0.254: IC5.27 62.5,90.23 62.5,92.25 57.75,97 22,97 17,92 17,87 15,85 J5.CONDUCTOR
N$32  (via drill 0.71)
  Top 0.4: R13.CCW 83.29,83.75 83.75,83.75 87,87 87,88.2 87.4,88.6 | IC6.7 C41.2 135.75,88.3 v135.75,89.5 | 87.4,88.6 C33.POS 88,89.2 88,91 90,93 PWR6.+VOUT 102.92,88.83 v103,88.75 | 87.4,88.6 85.92,90.08 IC5.15 77.89,91.89 79,93 C34.2 | v103,83 109,89 v111,89
  Bottom 0.4: v103,88.75 v103,83 | v111,89 135.25,89 v135.75,89.5
N$33
  Top 0.254: IC5.13 76.19,80.19 74.25,78.25 74.25,76 76,74.25 97,74.25 107.75,85 R15.1
N$34
  Top 0.254: R14.1 R18.2 77.89,77.06 IC5.14
N$35
  Top 0.254: R13.W 80.73,80.27 82,79 82,77.05 R14.2
N$36
  Top 0.178: IC2.7 136.95,59 R28.2 C58.2 139,59.75 140.25,61 140.25,61.98 SW2.2
N$37
  Bottom 0.18: 0,1 0,0 1,0
N$38
  Top 0.254: R15.2 121.5,85 | 121.5,85 R16.1 | C39.1 122.75,91 121.5,89.75 121.5,85
N$39
  Top 0.254: R16.2 124.95,86.5 | 124.95,86.5 C40.2 | IC6.3 125.18,86.73 124.95,86.5
N$40
  Top 0.178: 134.52,86.73 138.25,83 R17.1
  Top 0.254: 134.52,86.73 IC6.6 131.77,86.73 130.5,88 IC6.2 127.75,88 127,88.75 127,89.95 C39.2 | 148,83.05 R17.1
N$41  (via drill 0.71)
  Top 0.4: IC6.4 128.97,83.02 C42.2 129.2,83.25 v130.25,83.25 | C35.2 75.7,91 IC5.16 | 105.46,94.46 PWR6.TRM 105.46,88.21 102.25,85 92.8,85 C36.NEG | 105.46,94.46 107,96 112,96 113,95 113,93.08 PWR6.-VOUT 113.08,87.42 v113.5,87 | R13.CW 83.23,86.27 82,87.5 77.75,87.5 76.75,88.5 76.75,89.95 IC5.16 | 105.46,94.46 103.92,96 77.54,96 76.62,95.08 IC5.16
  Bottom 0.4: v113.5,87 126.5,87 v130.25,83.25
N$42
  Top 0.254: R17.2 150.25,83 152.25,85 J6.CONDUCTOR
N$43
  Top 0.4: C44.2 61.14,110.19 IC7.1 52.57,119 C43.POS 52.2,120.05 46.5,125.75 26,125.75 25,124.75 25,123.08 PWR7.+VOUT
N$44
  Top 0.4: IC7.2 62.86,110.19 C45.2 61.8,106.75 56.5,106.75 53.25,110 C46.NEG 52.2,110.8 49.5,113.5 43.5,113.5 35,122 | 27.46,123.46 PWR7.TRM 27.46,122.54 30.5,119.5 33,119.5 35,121.5 35,122 | 35,122 35,122.92 PWR7.-VOUT
N$45
  Top 0.254: IC7.27 62.5,120.23 62.5,122.25 57.75,127 22,127 17,122 17,117 15,115 J7.CONDUCTOR
N$46  (via drill 0.71)
  Top 0.4: R19.CCW 83.29,113.75 83.75,113.75 87,117 87,118.2 87.4,118.6 | IC8.7 C55.2 135.75,118.3 v135.75,119.5 | 87.4,118.6 C47.POS 88,119.2 88,121 90,123 PWR8.+VOUT 102.92,118.83 v103,118.75 | 87.4,118.6 85.92,120.08 IC7.15 77.89,121.89 79,123 C48.2
  Bottom 0.4: v103,118.75 135,118.75 v135.75,119.5
N$47
  Top 0.254: IC7.13 76.19,110.19 74.25,108.25 74.25,106 76,104.25 97,104.25 107.75,115 R21.1
N$48
  Top 0.254: R20.1 R24.2 77.89,107.06 IC7.14
N$49
  Top 0.254: R19.W 80.73,110.27 82,109 82,107.05 R20.2
N$50
  Bottom 0.18: 166,0 167,0 167,1
N$51
  Bottom 0.18: 166,140.75 167,140.75 167,139.6
N$52
  Top 0.254: R21.2 121.5,115 | 121.5,115 R22.1 | C53.1 122.75,121 121.5,119.75 121.5,115
N$53
  Top 0.254: R22.2 124.95,116.5 | 124.95,116.5 C54.2 | IC8.3 125.18,116.73 124.95,116.5
N$54
  Top 0.178: 134.52,116.73 138.25,113 R23.1
  Top 0.254: 134.52,116.73 IC8.6 131.77,116.73 130.5,118 IC8.2 127.75,118 127,118.75 127,119.95 C53.2
N$55  (via drill 0.71)
  Top 0.4: IC8.4 128.97,113.02 C56.2 129.2,113.25 v130.25,113.25 | C49.2 75.7,121 IC7.16 | 105.46,124.46 PWR8.TRM 105.46,118.21 102.25,115 92.8,115 C50.NEG | 105.46,124.46 107,126 112,126 113,125 113,123.08 PWR8.-VOUT 113.08,117.42 v113.5,117 | R19.CW 83.23,116.27 82,117.5 77.75,117.5 76.75,118.5 76.75,119.95 IC7.16 | 105.46,124.46 103.92,126 77.54,126 76.62,125.08 IC7.16
  Bottom 0.4: v113.5,117 126.5,117 v130.25,113.25
N$56
  Top 0.254: R23.2 150.25,113 152.25,115 J8.CONDUCTOR
N$57
  Bottom 0.18: 1,140.75 0,140.75 0,139.75
N$58
  Top 0.18: 77.5,0.25 77.5,4.5 arc-180 89.25,4.5 89.25,0.25
N$59
  Top 0.178: C57.1 R26.1 136.95,27 136.25,27 135.52,27.73 IC9.6 133.02,27.73 132.5,28.25 132.5,31.8 R25.1
N$60
  Top 0.18: 77.5,140.5 77.5,136.25 arc180 89.5,136.25 89.5,140.5
N$61
  Top 0.178: IC9.7 136.95,29 R26.2 C57.2 140.28,30.23 SW1.2
N$62
  Top 0.178: SW1.COM 143.22,28.77 147,25 R6.1
N$63
  Top 0.178: SW2.COM 143.47,58.77 147.25,55 R11.1
N$64
  Top 0.18: 0,139.75 0,140.75 1,140.75
N$65
  Top 0.18: 0,1 0,0 1,0

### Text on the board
Top: University of Toronto | Quad Analog Isolator 2 | Rev:A | J. Thywissen Labs | + | - | + | - | 0.5A | 12V+ | 12V-
Document: Quad Analog Isolator 2 | A. Stummer Oct '12 | A | 0.18mm | 0.5mm | 0.18mm | 0.25mm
